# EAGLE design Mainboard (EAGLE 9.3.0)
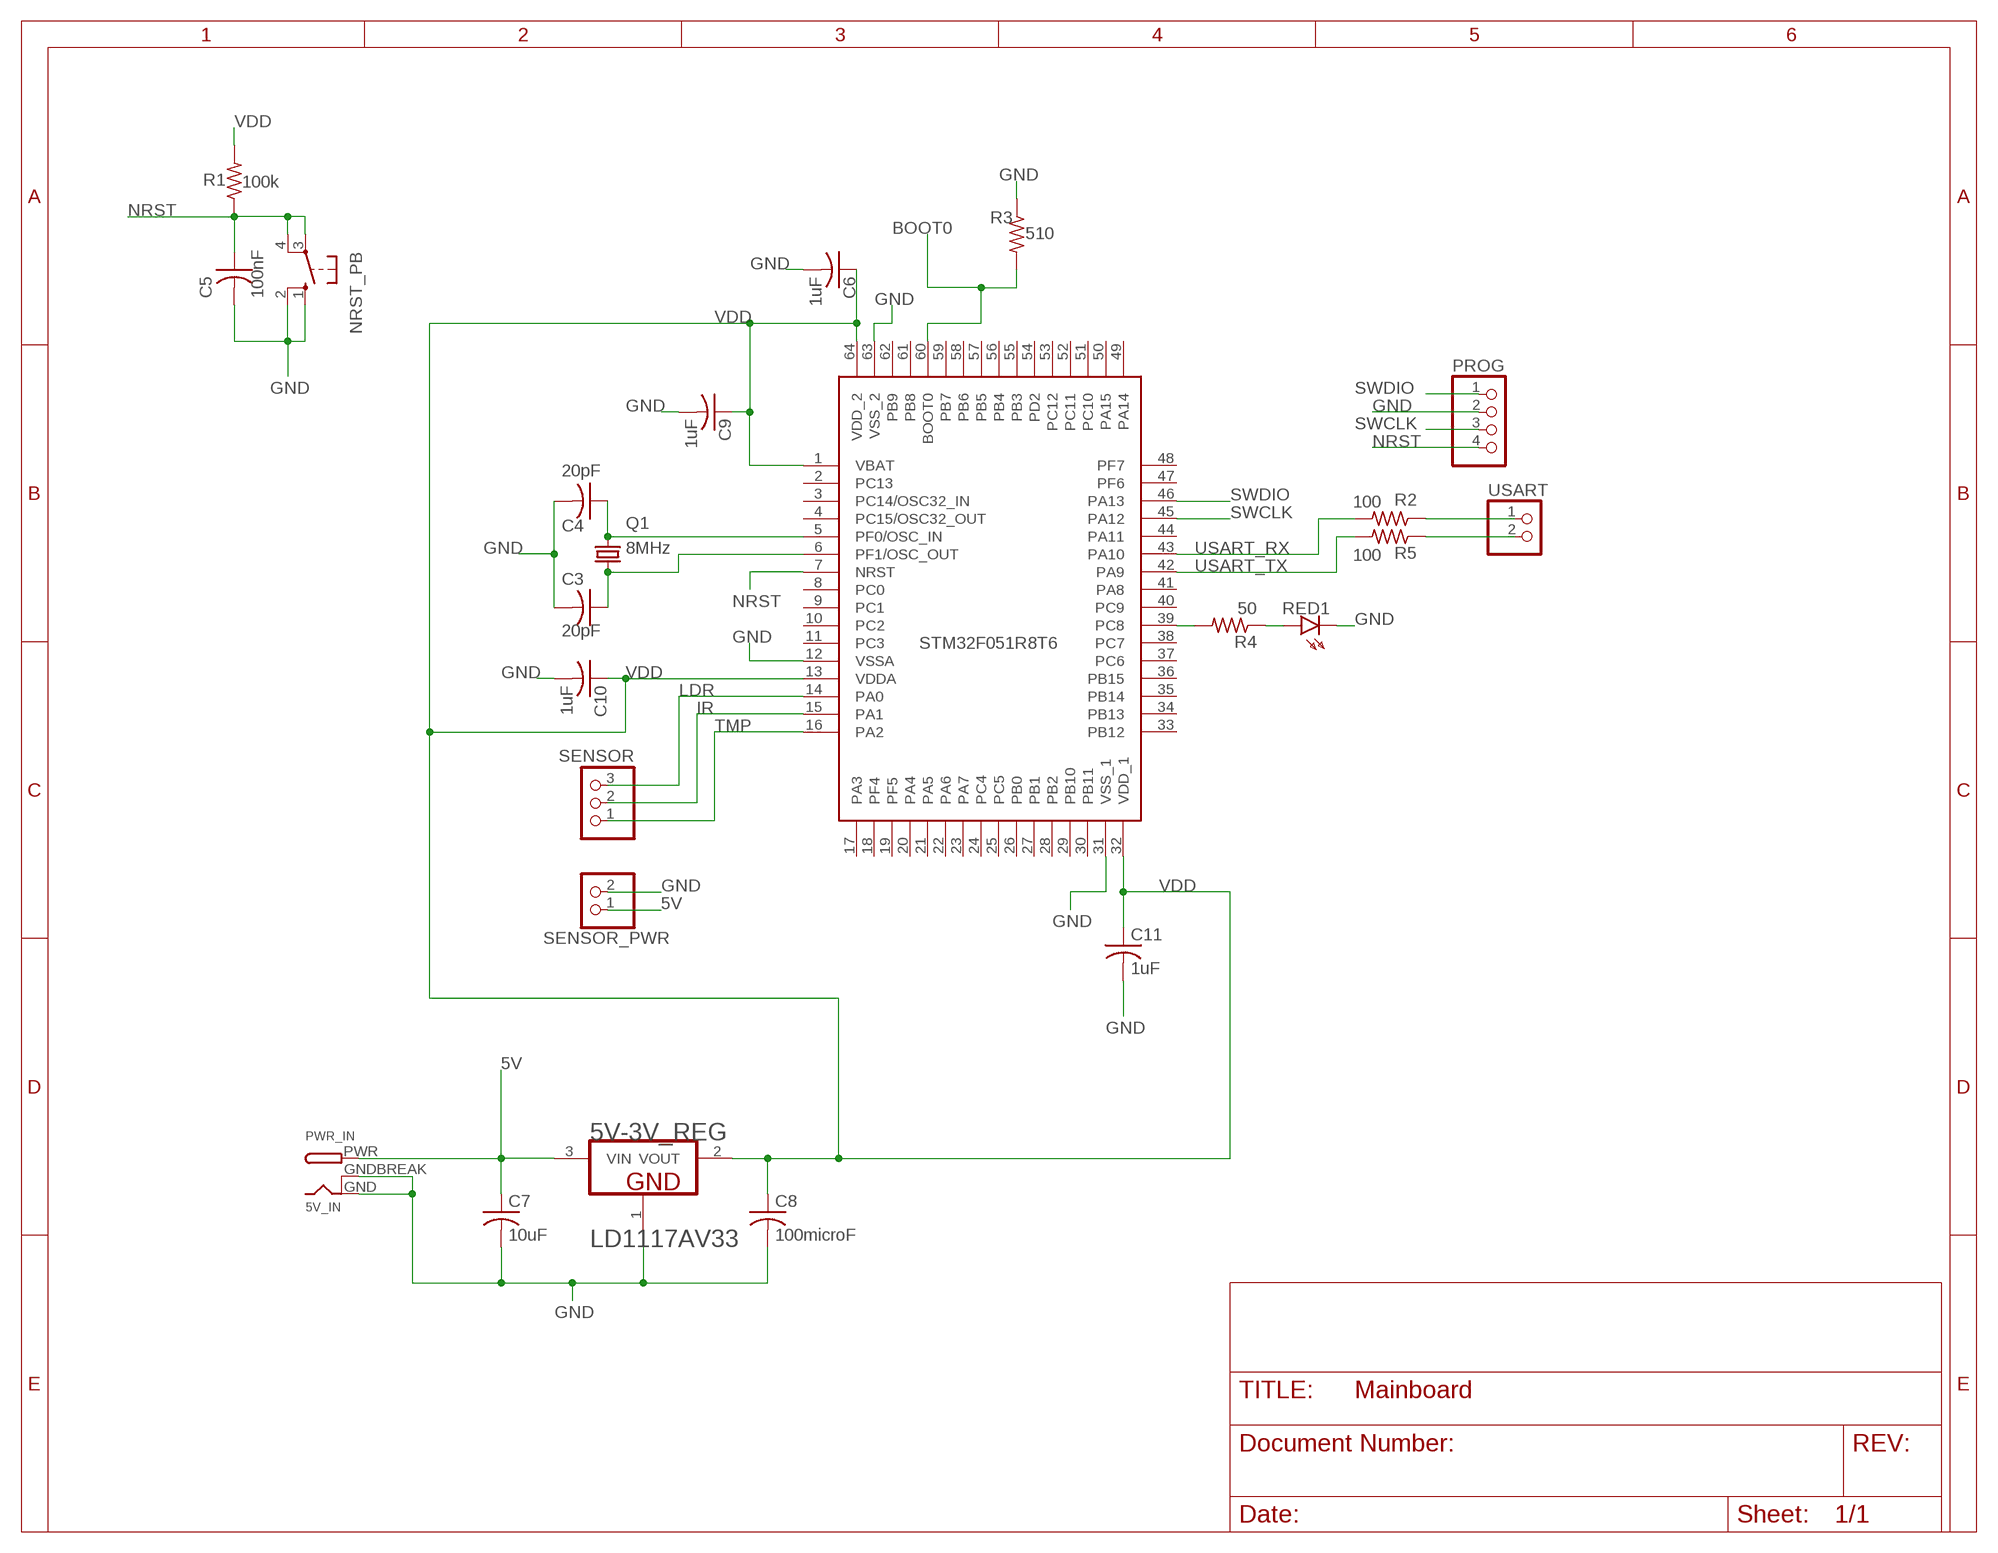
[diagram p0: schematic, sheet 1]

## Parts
5V-3V_REG  STMICROELECTRONICS_LD1117AV33STMICROELECTRONICS_LD1117AV33_0_0  [STMICROELECTRONICS_LD1117AV33_0]
C3  20pF  C-USC1206  [C1206]
C4  20pF  C-USC1206  [C1206]
C5  100nF  C-USC1206  [C1206]
C6  1uF  C-USC0805  [C0805]
C7  10uF  C-USC1206  [C1206]
C8  100microF  C-USC1206  [C1206]
C9  1uF  C-USC0805  [C0805]
C10  1uF  C-USC0805  [C0805]
C11  1uF  C-USC0805  [C0805]
IC1  STM32F051R8T6  [QFP50P1200X1200X160-64N]
JP2  SENSOR  PINHD-1X3  [1X03]
NRST_PB  10-XX  [B3F-10XX]
PROG  PINHD-1X4  [1X04]
PWR_IN  5V_IN  DCBARRELPTH  [DCJACK_2MM_PTH]
Q1  8MHz  CRYSTALHC49U-V  [HC49U-V]
R1  100k  R-US_0204/5  [0204/5]
R2  100  R-US_0204/5  [0204/5]
R3  510  R-US_0204/5  [0204/5]
R4  50  R-US_0204/5  [0204/5]
R5  100  R-US_0204/5  [0204/5]
RED1  HLMP6  [HLMP6]
SENSOR_PWR  PINHD-1X2  [1X02]
USART  PINHD-1X2  [1X02]

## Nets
5V: 5V-3V_REG.3(VIN) C7.1 PWR_IN.PWR SENSOR_PWR.1
BOOT0: IC1.60(BOOT0) R3.2
GND: 5V-3V_REG.1(GND) C3.2 C4.2 C5.2 C6.2 C7.2 C8.2 C9.2 C10.2 C11.2 IC1.12(VSSA) IC1.31(VSS_1) IC1.63(VSS_2) NRST_PB.1(S) NRST_PB.2(S1) PROG.2 PWR_IN.GND PWR_IN.GNDBREAK R3.1 RED1.K SENSOR_PWR.2
IR: IC1.15(PA1) JP2.2
LDR: IC1.14(PA0) JP2.3
N$3: IC1.39(PC8) R4.2
N$5: C3.1 IC1.6(PF1/OSC_OUT) Q1.2
N$6: R4.1 RED1.A
N$7: C4.1 IC1.5(PF0/OSC_IN) Q1.1
NRST: C5.1 IC1.7(NRST) NRST_PB.3(P) NRST_PB.4(P1) PROG.4 R1.1
SWCLK: IC1.45(PA12) PROG.3
SWDIO: IC1.46(PA13) PROG.1
TMP: IC1.16(PA2) JP2.1
USART_RX: IC1.43(PA10) R2.2
USART_RX1: R2.1 USART.1
USART_TX: IC1.42(PA9) R5.2
USART_TX1: R5.1 USART.2
VDD: 5V-3V_REG.2(VOUT) C6.1 C8.1 C9.1 C10.1 C11.1 IC1.1(VBAT) IC1.13(VDDA) IC1.32(VDD_1) IC1.64(VDD_2) R1.2
Unconnected: IC1.2(PC13) IC1.3(PC14/OSC32_IN) IC1.4(PC15/OSC32_OUT) IC1.8(PC0) IC1.9(PC1) IC1.10(PC2) IC1.11(PC3) IC1.17(PA3) IC1.18(PF4) IC1.19(PF5) IC1.20(PA4) IC1.21(PA5) IC1.22(PA6) IC1.23(PA7) IC1.24(PC4) IC1.25(PC5) IC1.26(PB0) IC1.27(PB1) IC1.28(PB2) IC1.29(PB10) IC1.30(PB11) IC1.33(PB12) IC1.34(PB13) IC1.35(PB14) IC1.36(PB15) IC1.37(PC6) IC1.38(PC7) IC1.40(PC9) IC1.41(PA8) IC1.44(PA11) IC1.47(PF6) IC1.48(PF7) IC1.49(PA14) IC1.50(PA15) IC1.51(PC10) IC1.52(PC11) IC1.53(PC12) IC1.54(PD2) IC1.55(PB3) IC1.56(PB4) IC1.57(PB5) IC1.58(PB6) IC1.59(PB7) IC1.61(PB8) IC1.62(PB9)

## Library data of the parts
5V-3V_REG = STMicroelectronics - LD1117AV33:STMICROELECTRONICS_LD1117AV33: PM-REG-LD1117V-SIL3; CIIVA_IDS: 1170378; COMPONENT_LINK_1_DESCRIPTION: Manufacturer URL; COMPONENT_LINK_1_URL: http://www.st.com; COMPONENT_LINK_3_DESCRIPTION: Package Specification; COMPONENT_LINK_3_URL: http://www.st.com/internet/com/TECHNICAL_RESOURCES/TECHNICAL_LITERATURE/PACKAGE_INFORMATION/CD00004649.pdf; DATASHEET: http://www.st.com/internet/com/TECHNICAL_RESOURCES/TECHNICAL_LITERATURE/DATASHEET/CD00002116.pdf; DATASHEET_VERSION: 2/12/2011; FOOTPRINT_VARIANT_NAME_0: Manufacturer Recommended; IMPORTED: yes; IMPORTED_FROM: vault; IMPORT_TS: 1521848985; MF: STMicroelectronics; MPN: LD1117AV33; PACKAGE: TO220; PACKAGE_DESCRIPTION: TO, Thru-Hole, Vertical, Heatsink Mounted; 3 In-Line Leads; Pitch 2.54 mm; PACKAGE_VERSION: ver3.0; PREFIX: U; RELEASE_DATE: 1329864168; VAULT_GUID: F0D7F0FA-C8CA-400E-8648-C9ECCD49760F; VAULT_REVISION: C5CAB179-AF12-4D57-B460-C843E566AF67
C3 C4 C6 C9-C11 = adafruit:C-US: CAPACITOR, American symbol
C5 C7 C8 = rcl:C-US: CAPACITOR, American symbol; SPICEPREFIX: C
IC1 = STMicroelectronics - STM32F051R8T6:STM32F051R8T6: Source: Datasheet; ALLIED_NUMBER: 70390941; ALLIED_PRICE-STOCK: http://www.alliedelec.com/stmicroelectronics-stm32f051r8t6/70390941/; HEIGHT: 1.6mm; MANUFACTURER_NAME: STMicroelectronics; MANUFACTURER_PART_NUMBER: STM32F051R8T6; MOUSER_PART_NUMBER: 511-STM32F051R8T6; MOUSER_PRICE-STOCK: https://www.mouser.com/Search/Refine.aspx?Keyword=511-STM32F051R8T6; RS_PART_NUMBER: 7618683P; RS_PRICE-STOCK: http://uk.rs-online.com/web/p/products/7618683P
JP2 = pinhead:PINHD-1X3: PIN HEADER
NRST_PB = switch-omron:10-XX: OMRON SWITCH; MPN: B3F-1000; OC_FARNELL: 176432; OC_NEWARK: 36M3542
PROG = pinhead:PINHD-1X4: PIN HEADER
PWR_IN = adafruit:DCBARREL: 2.0mm DC Barrel Jack DCJACK_2MM_PTH - Through Hole Jack (4UConnector: 05537)
Q1 = adafruit:CRYSTAL: CRYSTAL; OC_FARNELL: 1666969; OC_NEWARK: unknown
R1-R5 = adafruit:R-US_: RESISTOR, American symbol
RED1 = display-hp:HLMP6: LED; MF: AGILENT TECHNOLOGIES; MPN: HLMP-6500; OC_FARNELL: 1652490; OC_NEWARK: 40K0088
SENSOR_PWR USART = pinhead:PINHD-1X2: PIN HEADER

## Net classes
0 default: width 0.203 mm
3 gnd: width 0.508 mm

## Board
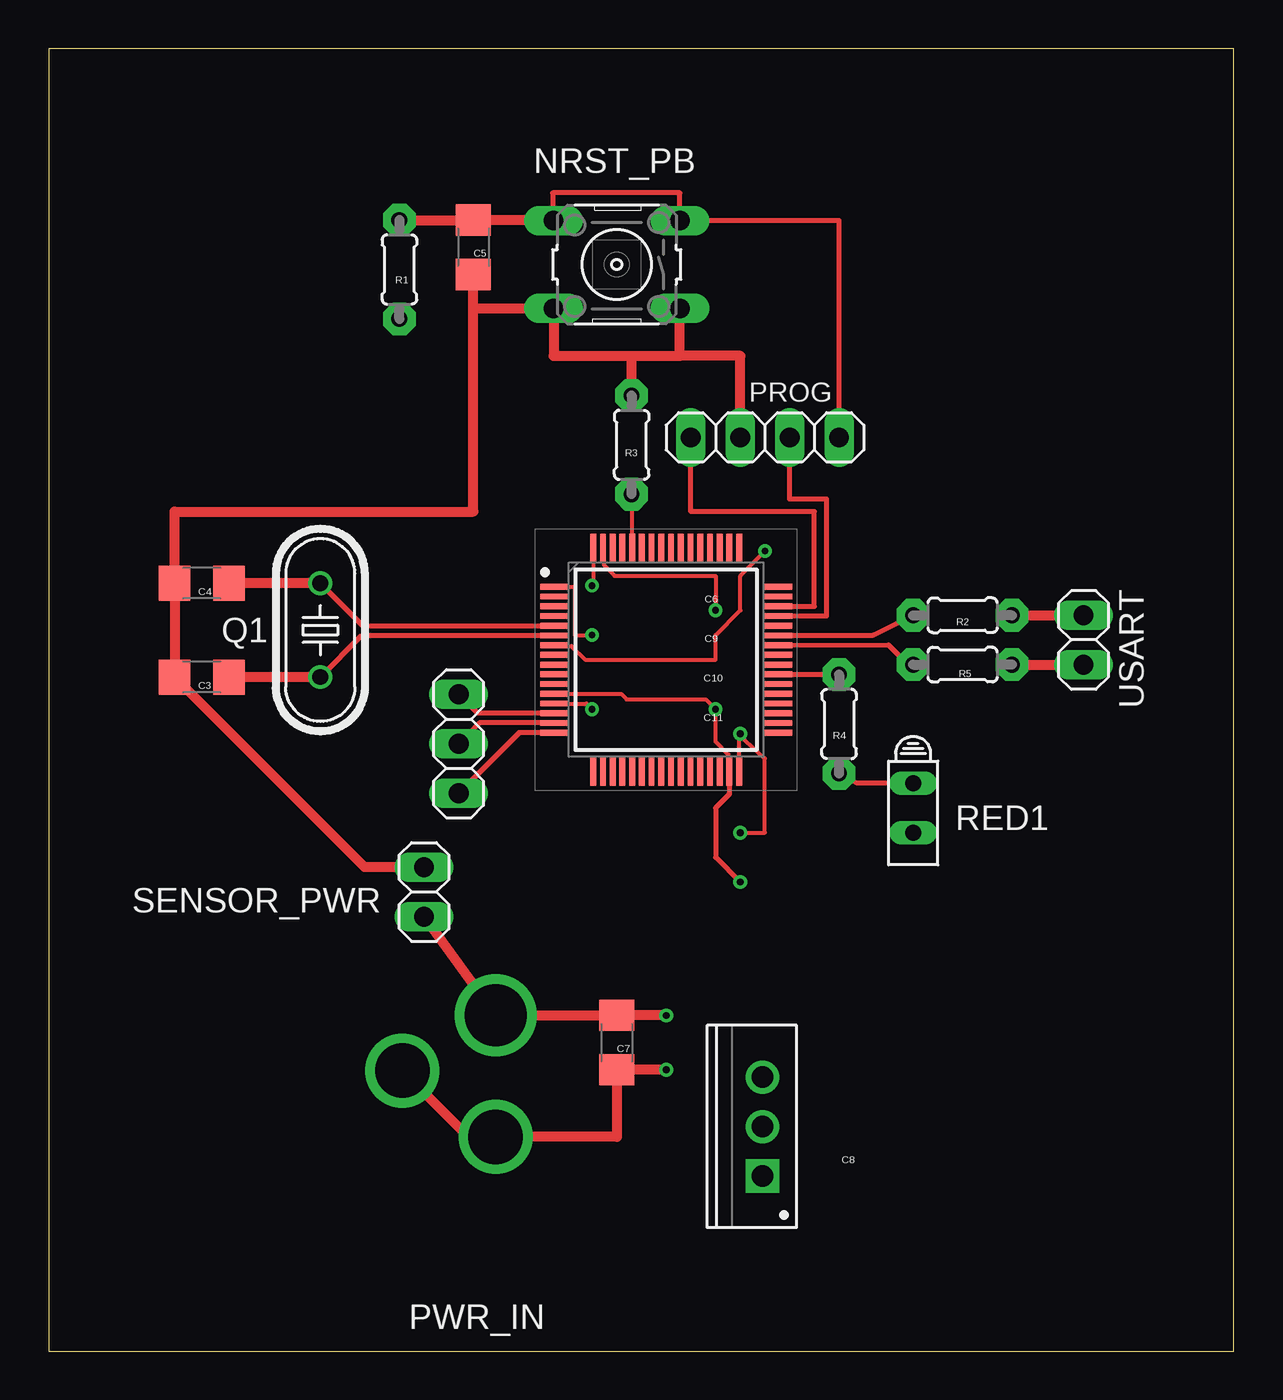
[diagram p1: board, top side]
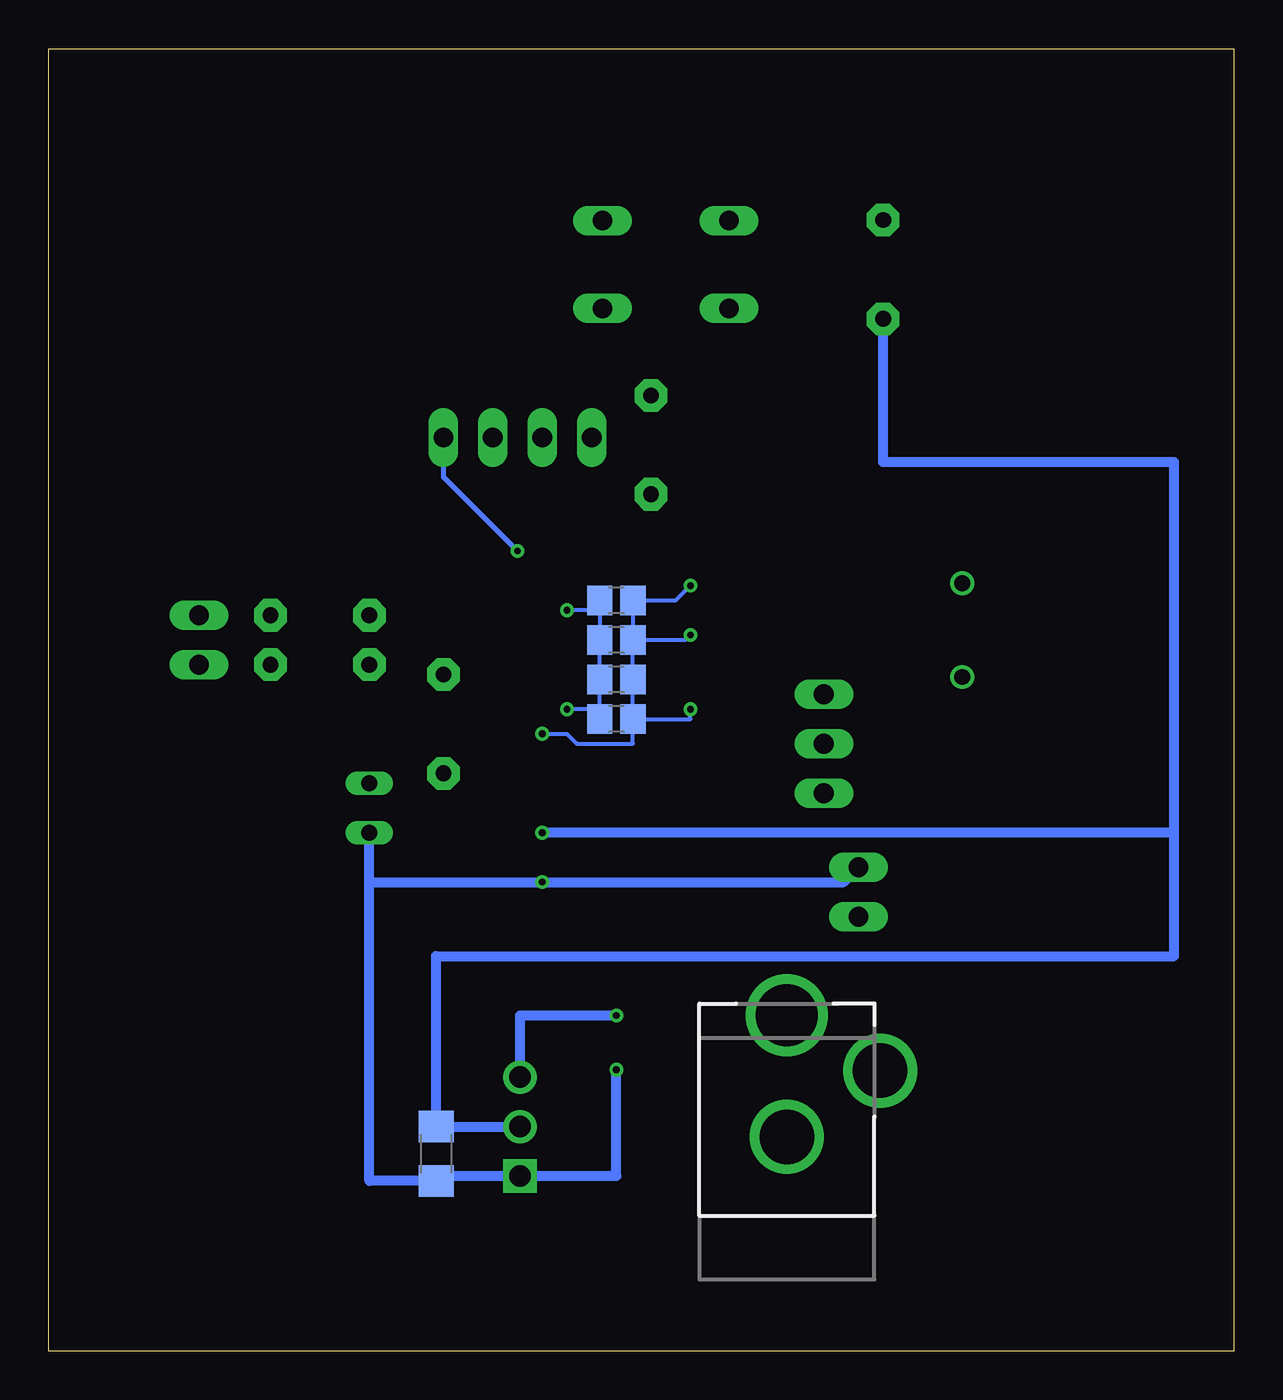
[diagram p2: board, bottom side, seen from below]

Size 60.94 x 66.98 mm. Coordinates in mm from the lower left corner, seen from the top.
Outline: 0,0 60.94,0 60.94,66.98 0,66.98 0,0
Copper layers (1*16): Top 0.0356mm / dielectric 1.5011mm / Bottom 0.0356mm
Design rules "ECE_Senior_Design": minimum track width 8mil, minimum drill 13mil, track to track 8mil, track to pad 8mil, pad to pad 6mil, via to via 8mil, smd to smd 6mil, copper to edge 15mil, drill to drill 8mil, minimum pad ring 7mil, minimum via ring 7mil, stop-mask expansion 3mil, vias tented up to drill 0mil, thermal gap 10mil

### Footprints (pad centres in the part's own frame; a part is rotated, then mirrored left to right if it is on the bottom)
STMICROELECTRONICS_LD1117AV33_0 = drill 1.1 pad 1.7 square: 1 -2.54,0 | drill 1.1 pad 1.7: 2 0,0; 3 2.54,0
C1206 = smd 1.6 x 1.8: 1 -1.4,0; 2 1.4,0
C0805 = smd 1.3 x 1.5: 1 -0.85,0; 2 0.85,0
QFP50P1200X1200X160-64N = smd 1.475 x 0.3: 1 -5.738,3.75; 2 -5.738,3.25; 3 -5.738,2.75; 4 -5.738,2.25; 5 -5.738,1.75; 6 -5.738,1.25; 7 -5.738,0.75; 8 -5.738,0.25; 9 -5.738,-0.25; 10 -5.738,-0.75; 11 -5.738,-1.25; 12 -5.738,-1.75; 13 -5.738,-2.25; 14 -5.738,-2.75; 15 -5.738,-3.25; 16 -5.738,-3.75; 33 5.738,-3.75; 34 5.738,-3.25; 35 5.738,-2.75; 36 5.738,-2.25; 37 5.738,-1.75; 38 5.738,-1.25; 39 5.738,-0.75; 40 5.738,-0.25; 41 5.738,0.25; 42 5.738,0.75; 43 5.738,1.25; 44 5.738,1.75; 45 5.738,2.25; 46 5.738,2.75; 47 5.738,3.25; 48 5.738,3.75 | smd 0.3 x 1.475: 17 -3.75,-5.738; 18 -3.25,-5.738; 19 -2.75,-5.738; 20 -2.25,-5.738; 21 -1.75,-5.738; 22 -1.25,-5.738; 23 -0.75,-5.738; 24 -0.25,-5.738; 25 0.25,-5.738; 26 0.75,-5.738; 27 1.25,-5.738; 28 1.75,-5.738; 29 2.25,-5.738; 30 2.75,-5.738; 31 3.25,-5.738; 32 3.75,-5.738; 49 3.75,5.738; 50 3.25,5.738; 51 2.75,5.738; 52 2.25,5.738; 53 1.75,5.738; 54 1.25,5.738; 55 0.75,5.738; 56 0.25,5.738; 57 -0.25,5.738; 58 -0.75,5.738; 59 -1.25,5.738; 60 -1.75,5.738; 61 -2.25,5.738; 62 -2.75,5.738; 63 -3.25,5.738; 64 -3.75,5.738
1X03 = drill 1.016 long: 1 -2.54,0; 2 0,0; 3 2.54,0
B3F-10XX = drill 1.016 long: 1 -3.251,2.261; 2 3.251,2.261; 3 -3.251,-2.261; 4 3.251,-2.261
1X04 = drill 1.016 long: 1 -3.81,0; 2 -1.27,0; 3 1.27,0; 4 3.81,0
DCJACK_2MM_PTH = drill 2.8: GND 0,7.35; GNDBREAK 4.8,10.75 | drill 3.2: PWR 0,13.6
HC49U-V = drill 0.813: 1 -2.413,0; 2 2.413,0
0204/5 = drill 0.813 pad 1.676 octagon: 1 -2.54,0; 2 2.54,0
HLMP6 = drill 0.813 long: A -1.27,0; K 1.27,0
1X02 = drill 1.016 long: 1 -1.27,0; 2 1.27,0

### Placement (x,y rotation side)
5V-3V_REG  36.7,11.56 90 top
C3  7.87,34.67 180 top
C4  7.87,39.5 180 top
C5  21.84,56.77 270 top
C6  31.75,38.61 180 bottom
C7  29.21,15.87 270 top
C8  41.02,10.16 270 bottom
C9  31.75,36.58 180 bottom
C10  31.75,34.54 180 bottom
C11  31.75,32.51 180 bottom
IC1  31.75,35.56 0 top
JP2  21.08,31.24 90 top
NRST_PB  29.21,55.88 180 top
PROG  36.83,46.99 0 top
PWR_IN  22.99,3.68 0 bottom
Q1  13.97,37.08 270 top
R1  18.03,55.63 270 top
R2  46.99,37.85 180 top
R3  29.97,46.61 270 top
R4  40.64,32.26 90 top
R5  46.99,35.31 180 top
RED1  44.45,27.94 270 top
SENSOR_PWR  19.3,23.62 90 top
USART  53.21,36.58 270 top

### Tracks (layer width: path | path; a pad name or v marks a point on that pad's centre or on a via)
5V  (via drill 0.35)
  Top 0.508: SENSOR_PWR.1 PWR_IN.PWR 29.2,17.28 | 29.2,17.28 C7.1 | v31.75,17.27 C7.1 29.2,17.28
  Bottom 0.508: 5V-3V_REG.3 36.7,17.27 v31.75,17.27
BOOT0
  Top 0.203: IC1.60 30,44.07 R3.2
GND  (via drill 0.35)
  Top 0.203: IC1.31 34.96,29.87 34.96,30.69 34.29,31.35 v34.29,33.02 33.78,33.53 29.72,33.53 29.44,33.81 IC1.12 | IC1.63 28.54,41.25 28.54,40.43 29.1,39.88 34.29,39.88 v34.29,38.1 | C5.2 21.84,53.62
  Top 0.254: IC1.31 35,28.65 34.29,27.94 34.29,25.4 v35.56,24.13
  Top 0.508: PWR_IN.GNDBREAK 21.59,11.03 PWR_IN.GND 29.21,11.03 C7.2 v31.75,14.48 | SENSOR_PWR.2 16.25,24.89 C3.2 C4.2 6.47,43.18 21.84,43.18 C5.2 | 32.46,51.18 NRST_PB.1 | 29.97,51.18 25.96,51.18 NRST_PB.2 21.84,53.62 | 29.97,51.18 32.46,51.18 | RED1.K 44.36,26.58 | PROG.2 35.56,51.18 32.46,51.18 | R3.1 29.97,51.18
  Bottom 0.203: v34.29,33.02 33.11,33.02 C11.2 C10.2 C9.2 C6.2 33.11,38.1 v34.29,38.1
  Bottom 0.508: v31.75,14.48 31.75,9.02 5V-3V_REG.1 40.76,9.02 arc-90 C8.2 44.45,8.76 44.45,24.13 | 44.45,24.13 RED1.K | 44.45,24.13 v35.56,24.13 20.07,24.13 SENSOR_PWR.2
IR
  Top 0.254: IC1.15 22.15,32.31 21.59,31.75 JP2.2
LDR
  Top 0.254: IC1.14 22.05,32.81 JP2.3
N$3
  Top 0.254: R4.2 IC1.39
N$5
  Top 0.254: Q1.2 16.11,36.81 IC1.6
  Top 0.508: Q1.2 C3.1
N$6
  Top 0.254: RED1.A 41.57,29.21 R4.1
N$7
  Top 0.254: Q1.1 16.16,37.31 IC1.5
  Top 0.508: Q1.1 C4.1
NRST  (via drill 0.35)
  Top 0.203: IC1.7 26.06,36.27 26.88,36.27 27.58,35.56 34.29,35.56 34.29,36.83 35.56,38.1 35.56,39.88 v36.83,41.15
  Top 0.254: 25.91,58.14 25.91,59.56 32.46,59.56 NRST_PB.3 40.64,58.14 PROG.4
  Top 0.508: C5.1 | 25.91,58.17 25.91,58.14 NRST_PB.4 arc90 25.93,58.17 C5.1 | R1.1 C5.1
  Bottom 0.254: PROG.4 40.64,44.96 v36.83,41.15
SWCLK
  Top 0.254: IC1.45 40.01,37.81 40.01,43.81 38.1,43.81 PROG.3
SWDIO
  Top 0.254: IC1.46 39.37,38.31 39.37,43.18 33.02,43.18 PROG.1
TMP
  Top 0.254: IC1.16 24.19,31.81 JP2.1
USART_RX
  Top 0.254: IC1.43 42.41,36.83 R2.2
USART_RX1
  Top 0.508: R2.1 USART.1
USART_TX
  Top 0.254: IC1.42 43.18,36.32 43.9,35.6 R5.2
USART_TX1
  Top 0.508: R5.1 USART.2
VDD  (via drill 0.35)
  Top 0.203: 35.56,29.88 arc-90 IC1.32 35.5,31.69 | 26.06,33.27 IC1.13 27.65,33.31 v27.94,33.02 | 35.5,26.73 arc90 v35.56,26.67 36.83,26.67 36.83,30.48 35.5,31.69 | 26.06,39.27 IC1.1 27.05,39.31 27.05,36.83 v27.94,36.83 | 27.94,41.24 arc-90 IC1.64 28,39.43 arc-90 v27.94,39.37 | 35.5,31.69 v35.56,31.75
  Bottom 0.203: C9.1 C6.1 28.7,38.61 v27.94,39.37 | C9.1 C10.1 C11.1 | v35.56,31.75 34.29,31.75 33.78,31.24 30.9,31.24 C11.1 | C11.1 27.94,32.51 v27.94,33.02 | C9.1 28.19,36.58 v27.94,36.83
  Bottom 0.508: 3.07,26.67 3.07,45.72 18.03,45.72 R1.2 | 3.07,26.67 3.07,20.32 41.02,20.32 C8.1 5V-3V_REG.2 | 3.07,26.67 arc-90 3.07,26.67 v35.56,26.67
